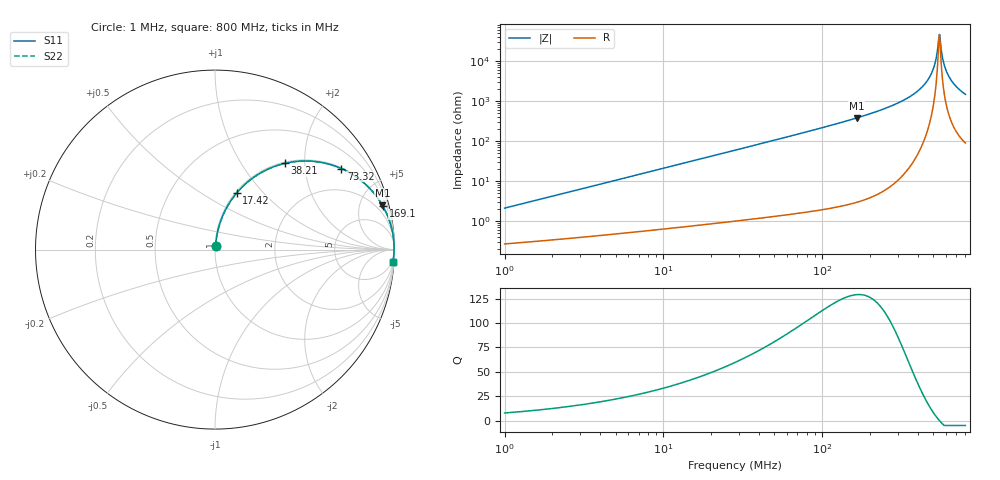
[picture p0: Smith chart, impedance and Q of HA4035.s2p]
# MHz S MA R 50
!Freq  MagS11  AngS11  MagS21  AngS21  MagS12  AngS12  MagS22  AngS22
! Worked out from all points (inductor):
!   801 points, 1 MHz to 800 MHz, reference 50 ohm
!   read as one part in series: L = 330 nH near 1.034 MHz
!   highest Q = 129 at 164.9 MHz (marker M1), where L = 363 nH
!   self-resonance near 544.7 MHz
!   S11 on the Smith chart (normalised r, x): 1 MHz: 1.01, +0.04; 17.42 MHz: 1.02, +0.72; 38.21 MHz: 1.02, +1.59; 73.32 MHz: 1.03, +3.10; 169.1 MHz: 1.06, +7.75; 800 MHz: 3, -29
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1  0.02084 81.5  0.9971 -1.2  0.9971 -1.2  0.02084 81.5
3.063851  0.06328 82.9  0.9941 -3.6  0.9941 -3.6  0.06328 82.9
9.30907  0.1886 77.3  0.9762 -10.9  0.9762 -10.9  0.1886 77.3
17.42092  0.3377 69.0  0.9339 -19.7  0.9339 -19.7  0.3377 69.0
28.28427  0.5033 58.8  0.8557 -30.2  0.8557 -30.2  0.5033 58.8
38.21062  0.6186 51.0  0.7769 -38.2  0.7769 -38.2  0.6186 51.0
73.32217  0.8361 32.7  0.5401 -56.7  0.5401 -56.7  0.8361 32.7
86.65878  0.8755 28.4  0.4751 -61.1  0.4751 -61.1  0.8755 28.4
164.9054  0.9645 14.9  0.2566 -74.7  0.2566 -74.7  0.9645 14.9
169.0914  0.9665 14.4  0.2495 -75.1  0.2495 -75.1  0.9665 14.4
263.3003  0.9889 8.0  0.1394 -81.4  0.1394 -81.4  0.9889 8.0
361.6996  0.9958 4.3  0.07509 -84.7  0.07509 -84.7  0.9958 4.3
445.7277  0.9977 2.1  0.03676 -85.4  0.03676 -85.4  0.9977 2.1
496.8723  0.998 1.0  0.01755 -82.9  0.01755 -82.9  0.998 1.0
513.76  0.998 0.7  0.01173 -79.8  0.01173 -79.8  0.998 0.7
535.679  0.9979 0.2  0.004713 -63.6  0.004713 -63.6  0.9979 0.2
549.2767  0.9978 -0.0  0.002159 4.3  0.002159 4.3  0.9978 -0.0
563.2196  0.9978 -0.3  0.005077 63.6  0.005077 63.6  0.9978 -0.3
592.1762  0.9975 -0.8  0.01357 79.0  0.01357 79.0  0.9975 -0.8
627.8458  0.9971 -1.4  0.0238 82.2  0.0238 82.2  0.9971 -1.4
699.8874  0.9959 -2.5  0.04309 83.3  0.04309 83.3  0.9959 -2.5
800  0.9936 -3.9  0.06746 82.7  0.06746 82.7  0.9936 -3.9
